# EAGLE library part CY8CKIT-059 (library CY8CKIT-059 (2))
CY8CKIT-059 PSoC® 5LP Prototyping Kit w/ CY8C5888LTI-LP097 Device Check availability
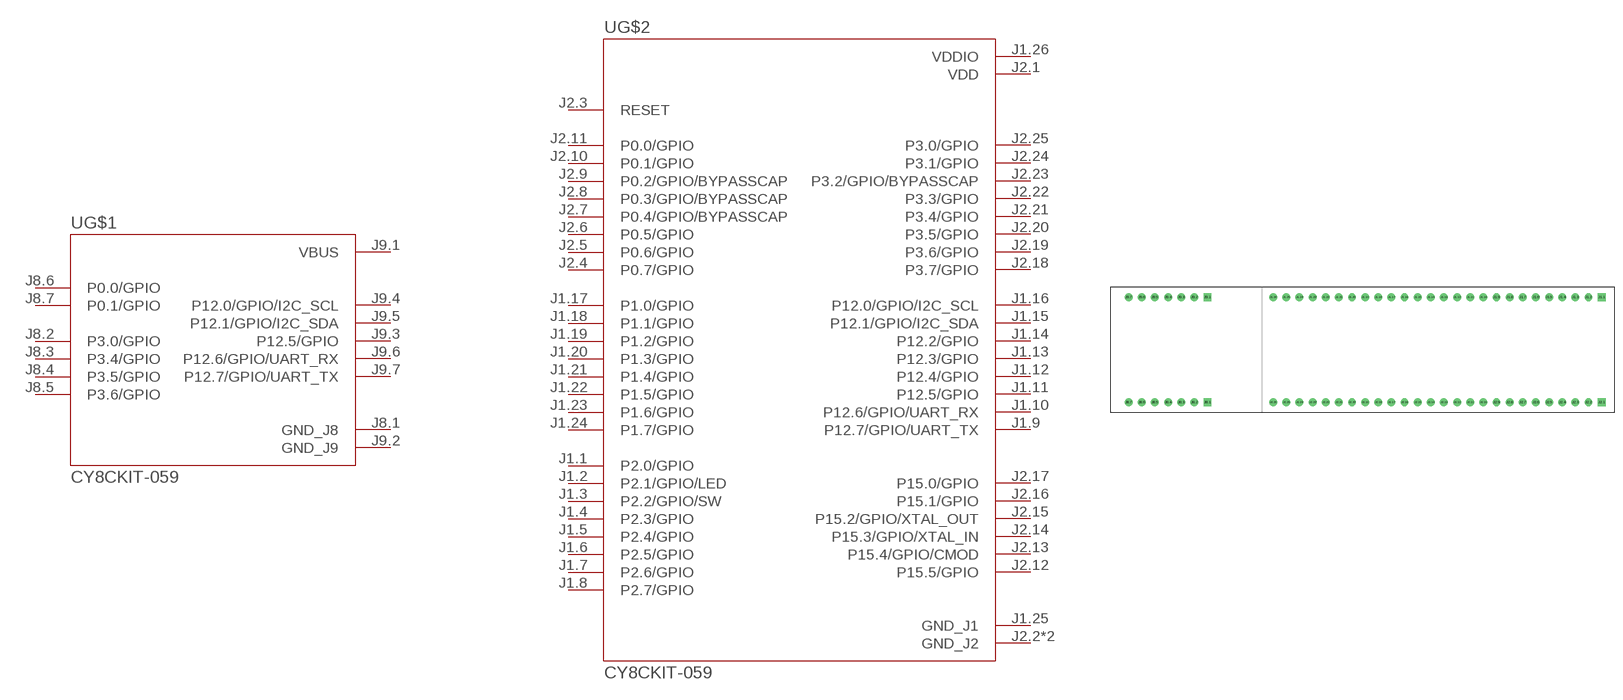
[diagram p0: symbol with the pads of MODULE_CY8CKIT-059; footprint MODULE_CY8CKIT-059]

Designator prefix U; gates G$1=CY8CKIT-059_KITPROG G$2=CY8CKIT-059_TARGET

## CY8CKIT-059 (Availability: In Stock; Check_prices: https://www.snapeda.com/parts/CY8CKIT-059/Cypress+semiconductor/view-part/?ref=eda; Description: CY8C58LP PSOC® 5LP ARM® Cortex®-M3 MCU 32-Bit Embedded Evaluation Board; MF: Cypress Semiconductor; MP: CY8CKIT-059; Package: None; Price: None; SnapEDA_Link: https://www.snapeda.com/parts/CY8CKIT-059/Cypress+semiconductor/view-part/?ref=snap)  [MODULE_CY8CKIT-059]
J1.1  G$2:P2.0/GPIO
J1.2  G$2:P2.1/GPIO/LED
J1.3  G$2:P2.2/GPIO/SW
J1.4  G$2:P2.3/GPIO
J1.5  G$2:P2.4/GPIO
J1.6  G$2:P2.5/GPIO
J1.7  G$2:P2.6/GPIO
J1.8  G$2:P2.7/GPIO
J1.9  G$2:P12.7/GPIO/UART_TX
J1.10  G$2:P12.6/GPIO/UART_RX
J1.11  G$2:P12.5/GPIO
J1.12  G$2:P12.4/GPIO
J1.13  G$2:P12.3/GPIO
J1.14  G$2:P12.2/GPIO
J1.15  G$2:P12.1/GPIO/I2C_SDA
J1.16  G$2:P12.0/GPIO/I2C_SCL
J1.17  G$2:P1.0/GPIO
J1.18  G$2:P1.1/GPIO
J1.19  G$2:P1.2/GPIO
J1.20  G$2:P1.3/GPIO
J1.21  G$2:P1.4/GPIO
J1.22  G$2:P1.5/GPIO
J1.23  G$2:P1.6/GPIO
J1.24  G$2:P1.7/GPIO
J1.25  G$2:GND_J1  pwr
J1.26  G$2:VDDIO  pwr
J2.1  G$2:VDD  pwr
J2.2  G$2:GND_J2  pwr
J2.3  G$2:RESET
J2.4  G$2:P0.7/GPIO
J2.5  G$2:P0.6/GPIO
J2.6  G$2:P0.5/GPIO
J2.7  G$2:P0.4/GPIO/BYPASSCAP
J2.8  G$2:P0.3/GPIO/BYPASSCAP
J2.9  G$2:P0.2/GPIO/BYPASSCAP
J2.10  G$2:P0.1/GPIO
J2.11  G$2:P0.0/GPIO
J2.12  G$2:P15.5/GPIO
J2.13  G$2:P15.4/GPIO/CMOD
J2.14  G$2:P15.3/GPIO/XTAL_IN
J2.15  G$2:P15.2/GPIO/XTAL_OUT
J2.16  G$2:P15.1/GPIO
J2.17  G$2:P15.0/GPIO
J2.18  G$2:P3.7/GPIO
J2.19  G$2:P3.6/GPIO
J2.20  G$2:P3.5/GPIO
J2.21  G$2:P3.4/GPIO
J2.22  G$2:P3.3/GPIO
J2.23  G$2:P3.2/GPIO/BYPASSCAP
J2.24  G$2:P3.1/GPIO
J2.25  G$2:P3.0/GPIO
J2.26  G$2:GND_J2  pwr
J8.1  G$1:GND_J8  pwr
J8.2  G$1:P3.0/GPIO
J8.3  G$1:P3.4/GPIO
J8.4  G$1:P3.5/GPIO
J8.5  G$1:P3.6/GPIO
J8.6  G$1:P0.0/GPIO
J8.7  G$1:P0.1/GPIO
J9.1  G$1:VBUS  pwr
J9.2  G$1:GND_J9  pwr
J9.3  G$1:P12.5/GPIO
J9.4  G$1:P12.0/GPIO/I2C_SCL
J9.5  G$1:P12.1/GPIO/I2C_SDA
J9.6  G$1:P12.6/GPIO/UART_RX
J9.7  G$1:P12.7/GPIO/UART_TX

## Footprint MODULE_CY8CKIT-059 (pad centres in mm)
drill 1.02 square: J1.1 45.72,10.16; J2.1 45.72,-10.16; J8.1 -30.48,-10.16; J9.1 -30.48,10.16
drill 1.02: J1.2 43.18,10.16; J1.3 40.64,10.16; J1.4 38.1,10.16; J1.5 35.56,10.16; J1.6 33.02,10.16; J1.7 30.48,10.16; J1.8 27.94,10.16; J1.9 25.4,10.16; J1.10 22.86,10.16; J1.11 20.32,10.16; J1.12 17.78,10.16; J1.13 15.24,10.16; J1.14 12.7,10.16; J1.15 10.16,10.16; J1.16 7.62,10.16; J1.17 5.08,10.16; J1.18 2.54,10.16; J1.19 0,10.16; J1.20 -2.54,10.16; J1.21 -5.08,10.16; J1.22 -7.62,10.16; J1.23 -10.16,10.16; J1.24 -12.7,10.16; J1.25 -15.24,10.16; J1.26 -17.78,10.16; J2.2 43.18,-10.16; J2.3 40.64,-10.16; J2.4 38.1,-10.16; J2.5 35.56,-10.16; J2.6 33.02,-10.16; J2.7 30.48,-10.16; J2.8 27.94,-10.16; J2.9 25.4,-10.16; J2.10 22.86,-10.16; J2.11 20.32,-10.16; J2.12 17.78,-10.16; J2.13 15.24,-10.16; J2.14 12.7,-10.16; J2.15 10.16,-10.16; J2.16 7.62,-10.16; J2.17 5.08,-10.16; J2.18 2.54,-10.16; J2.19 0,-10.16; J2.20 -2.54,-10.16; J2.21 -5.08,-10.16; J2.22 -7.62,-10.16; J2.23 -10.16,-10.16; J2.24 -12.7,-10.16; J2.25 -15.24,-10.16; J2.26 -17.78,-10.16; J8.2 -33.02,-10.16; J8.3 -35.56,-10.16; J8.4 -38.1,-10.16; J8.5 -40.64,-10.16; J8.6 -43.18,-10.16; J8.7 -45.72,-10.16; J9.2 -33.02,10.16; J9.3 -35.56,10.16; J9.4 -38.1,10.16; J9.5 -40.64,10.16; J9.6 -43.18,10.16; J9.7 -45.72,10.16

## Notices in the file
This work is licensed under a Creative Commons Attribution-ShareAlike 4.0 International License (CC BY-SA) with Design Exception 1.0
